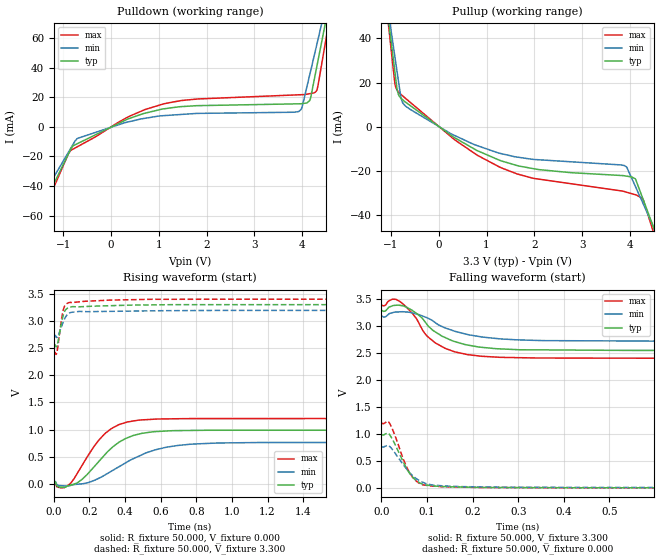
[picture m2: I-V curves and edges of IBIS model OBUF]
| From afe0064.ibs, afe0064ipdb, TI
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|   OBUF Model
[Model] OBUF
|Signals EOC(64), STO(63)
Model_type Output
Polarity   Non-Inverting
Enable   Active-Low
Vmeas = 1.65
Vref = 1.65
Cref = 0pF
Rref = 50
|output high   typ   min   max
|   (nom PVT)   (slow PVT)   (fast PVT)
|C_comp   3.3382980e-13   3.1674160e-13   3.4185980e-13
|output low   typ   min   max
|   (nom PVT)   (slow PVT)   (fast PVT)
 C_comp   4.7729290e-13   4.7457400e-13   5.1138920e-13
| Where   nom PVT is  Strong Process, 3.3V, 37C
|   Fast PVT is Nominal Process, 3.4V, 0C
|   Slow PVT is Weak Process, 3.2V, 95C
| variable   typ   min   max
[Voltage Range]   3.3   3.2   3.4
[Temperature Range]   37   95   0
|Operating temp range   27   85   0
[Pullup Reference]   3.3   3.2   3.4
[Pulldown Reference]   0   0   0
[Power Clamp Reference]   3.3   3.2   3.4
[GND Clamp Reference]   0   0   0
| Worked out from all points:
|   slope of the pulldown table from 0 to 0.495 V, typ, clamps not added: 69.4 ohm
|   slope of the pullup table from 0 to 0.495 V, typ, clamps not added: 69.2 ohm
|   falling waveform, R_fixture 50.000, V_fixture 3.300: 20-80 % time 78.2ps typ, 96.5ps min, 65.3ps max; typ from 3.3 V to 2.55 V
|   rising waveform, R_fixture 50.000, V_fixture 0.000: 20-80 % time 185ps typ, 273ps min, 161ps max; typ from 0 V to 0.991 V
|   rising waveform, R_fixture 50.000, V_fixture 3.300: 20-80 % time 29.4ps typ, 37.3ps min, 27.2ps max; typ from 2.55 V to 3.3 V
|   falling waveform, R_fixture 50.000, V_fixture 0.000: 20-80 % time 37.9ps typ, 46.3ps min, 34.9ps max; typ from 0.991 V to 0 V
[Pulldown]
|   Voltage   I(typ)   I(min)   I(max)
-3.3V     -181.1mA   -151.9mA   -198.7mA
-1.803V   -78.54mA   -67.01mA   -85.67mA
-893.4mV  -18.18mA   -17.08mA   -18.06mA
-702.9mV  -11.27mA   -7.743mA   -13.33mA
1.128V    12.36mA    7.704mA    15.83mA
3.926V    15.65mA    10.41mA    21.75mA
4.005V    15.81mA    14.3mA     21.86mA
4.168V    18.82mA    36.83mA    22.58mA
4.314V    42.16mA    56.9mA     25.56mA
4.452V    64.96mA    76.2mA     50.94mA
4.586V    87.16mA    94.78mA    76.14mA
6.59V     429.9mA    382.1mA    470.3mA
[Pullup]
|   Voltage   I(typ)   I(min)   I(max)
-3.3V     437.5mA    380.5mA    487.2mA
-1.498V   125.7mA    117mA      134.1mA
-927.7mV  26.33mA    32.95mA    21.14mA
-847.8mV  14.84mA    21.17mA    15.9mA
-787.7mV  12.85mA    12.91mA    14.63mA
-692.3mV  11.14mA    9.322mA    12.84mA
1.319V    -15.43mA   -12.12mA   -18.59mA
3.882V    -22.07mA   -17.44mA   -29.21mA
4.122V    -23.74mA   -27.19mA   -30.7mA
4.278V    -32.82mA   -34.71mA   -32.84mA
4.489V    -45.02mA   -44.89mA   -47.27mA
6.59V     -174mA     -153.7mA   -197.7mA
[Ramp]
R_load = 50
|   typ   min   max
dV/dt_r   0.594681/1.8394e-010   0.465412/2.70855e-010  0.723286/1.60002e-010
dV/dt_f   0.449493/7.69953e-011  0.289056/9.52199e-011   0.59632/6.46045e-011
[Falling Waveform]
R_fixture = 50.000
V_fixture = 3.300
V_fixture_min = 3.200
V_fixture_max = 3.400
C_fixture = 0.000
|  time   V(typ)   V(min)   V(max)
0s        3.3V       3.194V     3.4V
6.696ps   3.281V     3.175V     3.384V
24.35ps   3.383V     3.254V     3.506V
41.44ps   3.389V     3.271V     3.456V
68.24ps   3.292V     3.248V     3.237V
100.2ps   3.032V     3.159V     2.818V
138.8ps   2.796V     2.974V     2.595V
183.4ps   2.662V     2.86V      2.485V
257.5ps   2.583V     2.77V      2.426V
3.055ns   2.551V     2.724V     2.406V
[Rising Waveform]
R_fixture = 50.000
V_fixture = 0.000
V_fixture_min = 0.000
V_fixture_max = 0.000
C_fixture = 0.000
|  time   V(typ)   V(min)   V(max)
0s        -48.57pV   6.342mV    -244.9pV
59.09ps   -59.33mV   -34.99mV   -66.88mV
132.6ps   23.46mV    -4.176mV   200.7mV
226ps     316.5mV    65.17mV    691.7mV
290.3ps   552.3mV    172.5mV    935.8mV
369.8ps   776.2mV    325mV      1.097V
475.3ps   916.2mV    508.8mV    1.174V
633.3ps   974.8mV    676.9mV    1.197V
921.6ps   988.7mV    754mV      1.203V
3.055ns   991.1mV    765.3mV    1.205V
[Rising Waveform]
R_fixture = 50.000
V_fixture = 3.300
V_fixture_min = 3.200
V_fixture_max = 3.400
C_fixture = 0.000
|  time   V(typ)   V(min)   V(max)
0s        2.551V     2.724V     2.406V
4.474ps   2.566V     2.739V     2.426V
13.27ps   2.521V     2.699V     2.383V
17.44ps   2.54V      2.697V     2.423V
43.36ps   2.966V     2.898V     3.034V
55.28ps   3.128V     2.999V     3.228V
68.21ps   3.213V     3.084V     3.305V
88.61ps   3.25V      3.147V     3.34V
549ps     3.294V     3.185V     3.397V
3.055ns   3.3V       3.194V     3.4V
[Falling Waveform]
R_fixture = 50.000
V_fixture = 0.000
V_fixture_min = 0.000
V_fixture_max = 0.000
C_fixture = 0.000
|  time   V(typ)   V(min)   V(max)
0s        991.2mV    765.3mV    1.206V
13.21ps   1.019V     790.3mV    1.239V
18.16ps   984.7mV    768.3mV    1.194V
28.94ps   820.7mV    654.8mV    987mV
53.13ps   391.7mV    372.7mV    426.6mV
72.53ps   161.7mV    196.3mV    155.8mV
90.13ps   70.55mV    104.6mV    57.82mV
131.6ps   26.61mV    39.27mV    21.68mV
475.1ps   1.659mV    7.805mV    1.802mV
3.055ns   63.04uV    6.342mV    60.26uV
